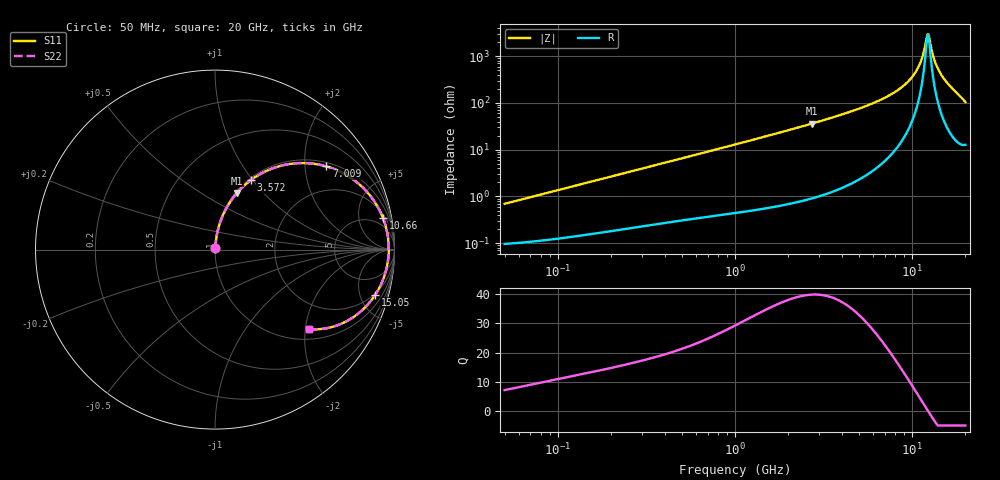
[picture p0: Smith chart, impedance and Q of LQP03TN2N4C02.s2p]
!Murata Part Number: LQP03TN2N4C02
!These Parameters are Measured in Series Mode Connection
!  o--[Z]--o
!Port1  Port2
!  o-------o
!Freq. Start=50[MHz] Stop=20[GHz], 401[Steps]
# Hz S RI R 50
!Freq.(Hz) S11(Real) S11(Imag) S21(Real) S21(Imag) S12(Real) S12(Imag) S22(Real) S22(Imag)
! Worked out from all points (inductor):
!   401 points, 50 MHz to 20 GHz, reference 50 ohm
!   read as one part in series: L = 2.19 nH near 51.52 MHz
!   highest Q = 39.9 at 2.728 GHz (marker M1), where L = 2.12 nH
!   self-resonance near 12.2 GHz
!   S11 on the Smith chart (normalised r, x): 50 MHz: 1.00, +0.01; 3.572 GHz: 1.03, +0.98; 7.009 GHz: 1.11, +2.58; 10.66 GHz: 3, +10; 15.05 GHz: 1.87, -6.75; 20 GHz: 1.25, -2.09
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5e7  0.00101 0.00688  0.999 -0.00688  0.999 -0.00688  0.00101 0.00688
1.364002e8  0.0018 0.0183  0.9982 -0.0183  0.9982 -0.0183  0.0018 0.0183
3.721004e8  0.00494 0.0484  0.9951 -0.0484  0.9951 -0.0484  0.00494 0.0484
1e9  0.0205 0.1257  0.9795 -0.1257  0.9795 -0.1257  0.0205 0.1257
2.728004e9  0.1226 0.3157  0.8774 -0.3157  0.8774 -0.3157  0.1226 0.3157
3.572216e9  0.2012 0.3882  0.7988 -0.3882  0.7988 -0.3882  0.2012 0.3882
4.966507e9  0.3611 0.4655  0.6389 -0.4655  0.6389 -0.4655  0.3611 0.4655
7.009217e9  0.6201 0.4638  0.3799 -0.4638  0.3799 -0.4638  0.6201 0.4638
7.442007e9  0.672 0.4457  0.328 -0.4457  0.328 -0.4457  0.672 0.4457
9.178299e9  0.8463 0.3221  0.1537 -0.3221  0.1537 -0.3221  0.8463 0.3221
1.004137e10  0.9061 0.2389  0.0939 -0.2389  0.0939 -0.2389  0.9061 0.2389
1.066139e10  0.9365 0.1743  0.0635 -0.1743  0.0635 -0.1743  0.9365 0.1743
1.131968e10  0.9575 0.1039  0.0425 -0.1039  0.0425 -0.1039  0.9575 0.1039
1.201863e10  0.9675 0.0292  0.0325 -0.0292  0.0325 -0.0292  0.9675 0.0292
1.238412e10  0.9681 -0.00902  0.0319 0.00902  0.0319 0.00902  0.9681 -0.00902
1.257102e10  0.9672 -0.0283  0.0328 0.0283  0.0328 0.0283  0.9672 -0.0283
1.314879e10  0.9597 -0.086  0.0403 0.086  0.0403 0.086  0.9597 -0.086
1.354865e10  0.9506 -0.1242  0.0494 0.1242  0.0494 0.1242  0.9506 -0.1242
1.417136e10  0.9309 -0.1802  0.0691 0.1802  0.0691 0.1802  0.9309 -0.1802
1.504638e10  0.8933 -0.251  0.1067 0.251  0.1067 0.251  0.8933 -0.251
1.696185e10  0.7791 -0.3706  0.2209 0.3706  0.2209 0.3706  0.7791 -0.3706
2e10  0.5219 -0.4422  0.4781 0.4422  0.4781 0.4422  0.5219 -0.4422
